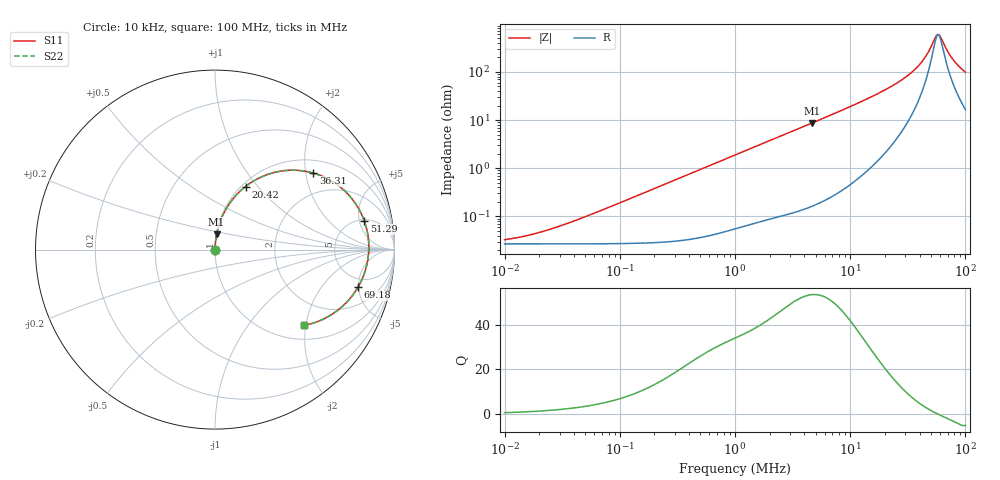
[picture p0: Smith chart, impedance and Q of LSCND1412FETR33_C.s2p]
! LSCND1412FETR33_C  S-PARAMETER MODEL  ( Standard Model )
! Model Generated by TAIYO YUDEN Corporation (http://www.ty-top.com)
! Version 1.0
! TAIYO YUDEN Control No. 201211
! Copyright(c) 2020 TAIYO YUDEN CO.,LTD. All Rights Reserved.
! Product Description (link to TY-COMPAS)
! https://ds.yuden.co.jp/TYCOMPAS/or/detail?pn=LSCND1412FETR33MC&u=M
! Products Name : Inductors
! Characteristics :
!  Inductance : 0.33 [uH] , SRF(min) : - [Hz] , DC Resistance(max) : 32 [mOhm]
!  Rated Current : Saturation  5.0 [A] (dL = 30 [%]), Temp Rise  3.7 [A] (dT = 40 [degC])
!  Case Size : 1.4 x 1.2 / 0.055 x 0.047 [mm/inch] , Thickness : 0.65 / 0.026 [mm/inch]
!  (Conditions: Temperature = 25 [degC] , DC Bias Current = 0 [A])
! External Node Assignments :
!  1  o---GGG---o  2
! GND o---------o GND
! Frequency Range : 10kHz  -  100MHz  [ 402 STEP ]
# MHz S RI R 50
! Freq[MHz].  S11 Real  S11 Imag  S21 Real  S21 Imag  S12 Real  S12 Imag  S22 Real  S22 Imag
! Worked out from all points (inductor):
!   401 points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, 10 kHz to 100 MHz, reference 50 ohm
!   read as one part in series: L = 302 nH near 43.65 kHz
!   highest Q = 53.4 at 4.677 MHz (marker M1), where L = 296 nH
!   self-resonance near 58.11 MHz
!   S11 on the Smith chart (normalised r, x): 10 kHz: 1.00, +0.00; 20.42 MHz: 1.04, +0.87; 36.31 MHz: 1.34, +2.21; 51.29 MHz: 5.24, +5.94; 69.18 MHz: 3.77, -4.92; 100 MHz: 1.33, -1.95
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0.01  0.000269 0.000189  0.9997 -0.000189  0.9997 -0.000189  0.000269 0.000189
0.019953  0.000269 0.000378  0.9997 -0.000378  0.9997 -0.000378  0.000269 0.000378
0.046774  0.000271 0.000886  0.9997 -0.000886  0.9997 -0.000886  0.000271 0.000886
0.218776  0.000306 0.00414  0.9997 -0.00414  0.9997 -0.00414  0.000306 0.00414
1  0.000904 0.0187  0.9991 -0.0187  0.9991 -0.0187  0.000904 0.0187
4.677351  0.0091 0.0861  0.9909 -0.0861  0.9909 -0.0861  0.0091 0.0861
11.74898  0.0541 0.213  0.9459 -0.213  0.9459 -0.213  0.0541 0.213
15.84893  0.0999 0.2823  0.9001 -0.2823  0.9001 -0.2823  0.0999 0.2823
20.41738  0.1701 0.3514  0.8299 -0.3514  0.8299 -0.3514  0.1701 0.3514
21.87762  0.1968 0.3708  0.8032 -0.3708  0.8032 -0.3708  0.1968 0.3708
28.18383  0.3352 0.431  0.6648 -0.431  0.6648 -0.431  0.3352 0.431
36.30781  0.5473 0.4265  0.4527 -0.4265  0.4527 -0.4265  0.5473 0.4265
43.65158  0.7218 0.3279  0.2782 -0.3279  0.2782 -0.3279  0.7218 0.3279
47.86301  0.7934 0.24  0.2066 -0.24  0.2066 -0.24  0.7934 0.24
51.28614  0.8318 0.16  0.1682 -0.16  0.1682 -0.16  0.8318 0.16
56.23413  0.8562 0.0425  0.1438 -0.0425  0.1438 -0.0425  0.8562 0.0425
58.88437  0.8561 -0.0175  0.1439 0.0175  0.1439 0.0175  0.8561 -0.0175
61.6595  0.8479 -0.0763  0.1521 0.0763  0.1521 0.0763  0.8479 -0.0763
69.1831  0.7967 -0.2094  0.2033 0.2094  0.2033 0.2094  0.7967 -0.2094
74.13102  0.7497 -0.2754  0.2503 0.2754  0.2503 0.2754  0.7497 -0.2754
81.28305  0.6754 -0.3443  0.3246 0.3443  0.3246 0.3443  0.6754 -0.3443
100  0.4946 -0.4227  0.5054 0.4227  0.5054 0.4227  0.4946 -0.4227
